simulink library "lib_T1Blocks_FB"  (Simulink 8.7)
settings: Solver=ode3  SolverMode=SingleTasking  StartTime=0.0  StopTime=1  FixedStep=0.02/16384  RelTol=1e-3
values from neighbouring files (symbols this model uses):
  Tstep = 0.0005    [TestOrthOscObjO_init.m]    (also in TestWaveMng_init.m = 5e-05)
undefined symbols (not defined in the file or in its folder): lim, max_error, min_decrease, min_reset, P_TA, T1, Td, y0
libraries: lib_T1Blocks_FB x7, simulink x2

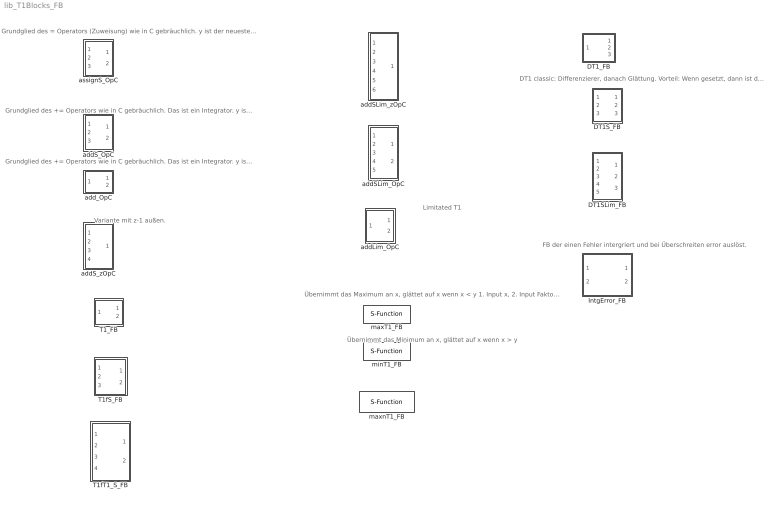
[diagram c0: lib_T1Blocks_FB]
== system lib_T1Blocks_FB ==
  note: Limitated T1
  note: Variante mit z-1 außen.
  note: Übernimmt das Maximum an x, glättet auf x wenn x < y 1. Input x, 2. Input Faktor zum Glätten
  note: DT1 classic: Differenzierer, danach Glättung. Vorteil: Wenn gesetzt, dann ist das Differnzial 0
  note: Grundglied des += Operators wie in C gebräuchlich. Das ist ein Integrator. y ist der neueste Wert. yz ist der gespeicherte Wert (Abarbeitung bevor +=). Setzen: Wird in C häufig an anderer Stelle ausgeführt.
  note: Grundglied des += Operators wie in C gebräuchlich. Das ist ein Integrator. y ist der neueste Wert. yz ist der gespeicherte Wert (Abarbeitung bevor +=). Ohne Setz-Möglichkeit. Initialwert als Parameter.
  note: FB der einen Fehler intergriert und bei Überschreiten error auslöst.
  note: Grundglied des = Operators (Zuweisung) wie in C gebräuchlich. y ist der neueste Wert, entweder =X oder =XS. yz ist der gespeicherte Wert. Setzen: Wird in C häufig an anderer Stelle ausgeführt.
  note: Übernimmt das Minimum an x, glättet auf x wenn x > y
  DT1SLim_FB : Subsystem
  DT1S_FB : Subsystem
  DT1_FB : Subsystem
  IntgError_FB : Subsystem
  T1_FB : Subsystem
  T1fS_FB : Subsystem
  T1fT1_S_FB : Subsystem
  addLim_OpC : Subsystem
  addSLim_OpC : Subsystem
  addSLim_zOpC : Subsystem
  addS_OpC : Subsystem
  addS_zOpC : Subsystem
  add_OpC : Subsystem
  assignS_OpC : Subsystem
  maxT1_FB : S-Function  FunctionName=maxT1_FB  Parameters=SampleTime  SFunctionDeploymentMode=off  EnableBusSupport=off
  maxnT1_FB : S-Function  FunctionName=maxnT1_FB  Parameters=SampleTime  SFunctionDeploymentMode=off  EnableBusSupport=off
  minT1_FB : S-Function  FunctionName=minT1_FB  Parameters=SampleTime  SFunctionDeploymentMode=off  EnableBusSupport=off

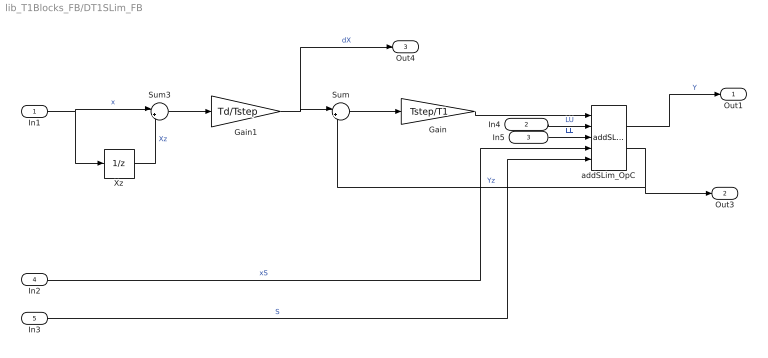
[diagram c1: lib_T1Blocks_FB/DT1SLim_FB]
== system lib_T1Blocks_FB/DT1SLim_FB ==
  In1 : Inport
  In4 : Inport  Port=2
  In5 : Inport  Port=3
  In2 : Inport  Port=4
  In3 : Inport  Port=5
  Gain : Gain  Gain=Tstep/T1
  Gain1 : Gain  Gain=Td/Tstep
  Sum : Sum  Inputs=|+-
  Sum3 : Sum  Inputs=|+-
  Xz : UnitDelay  SampleTime=-1
  addSLim_OpC : lib_T1Blocks_FB/addSLim_OpC
  Out1 : Outport
  Out3 : Outport  Port=2
  Out4 : Outport  Port=3
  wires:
  addSLim_OpC/2 -> Out3/1, Sum/2  "Yz"
  In3/1 -> addSLim_OpC/5  "S"
  In2/1 -> addSLim_OpC/4  "xS"
  Sum3/1 -> Gain1/1
  Xz/1 -> Sum3/2  "Xz"
  Gain1/1 -> Sum/1, Out4/1  "dX"
  addSLim_OpC/1 -> Out1/1  "Y"
  In1/1 -> Sum3/1, Xz/1  "x"
  Sum/1 -> Gain/1
  Gain/1 -> addSLim_OpC/1
  In4/1 -> addSLim_OpC/2  "LU"
  In5/1 -> addSLim_OpC/3  "LL"

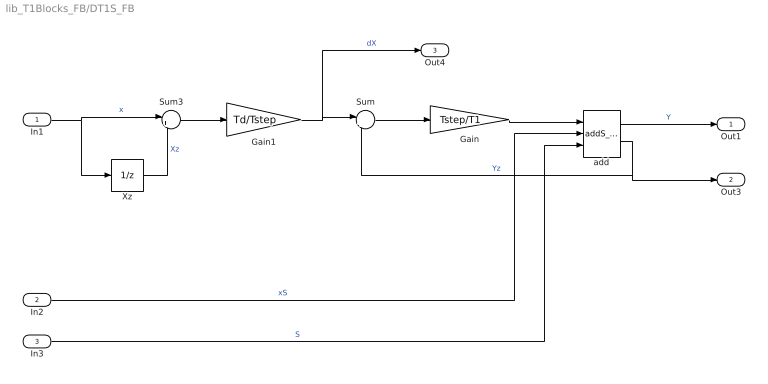
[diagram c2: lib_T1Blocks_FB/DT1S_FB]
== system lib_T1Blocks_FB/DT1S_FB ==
  In1 : Inport
  In2 : Inport  Port=2
  In3 : Inport  Port=3
  Gain : Gain  Gain=Tstep/T1
  Gain1 : Gain  Gain=Td/Tstep
  Sum : Sum  Inputs=|+-
  Sum3 : Sum  Inputs=|+-
  Xz : UnitDelay  SampleTime=-1
  add : lib_T1Blocks_FB/addS_OpC
  Out1 : Outport
  Out3 : Outport  Port=2
  Out4 : Outport  Port=3
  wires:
  Gain/1 -> add/1
  Sum/1 -> Gain/1
  In1/1 -> Xz/1, Sum3/1  "x"
  add/1 -> Out1/1  "Y"
  Gain1/1 -> Out4/1, Sum/1  "dX"
  Xz/1 -> Sum3/2  "Xz"
  Sum3/1 -> Gain1/1
  In2/1 -> add/2  "xS"
  In3/1 -> add/3  "S"
  add/2 -> Sum/2, Out3/1  "Yz"

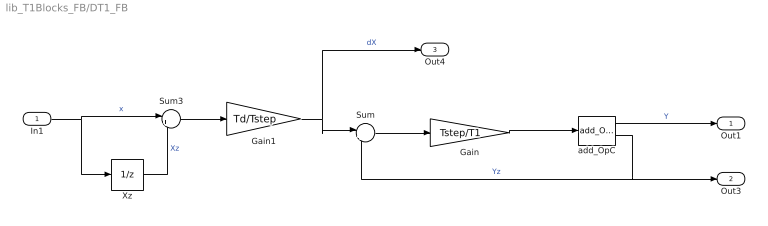
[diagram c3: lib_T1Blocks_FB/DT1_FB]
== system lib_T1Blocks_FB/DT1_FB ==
  In1 : Inport
  Gain : Gain  Gain=Tstep/T1
  Gain1 : Gain  Gain=Td/Tstep
  Sum : Sum  Inputs=|+-
  Sum3 : Sum  Inputs=|+-
  Xz : UnitDelay  SampleTime=-1
  add_OpC : lib_T1Blocks_FB/add_OpC  y0=0
  Out1 : Outport
  Out3 : Outport  Port=2
  Out4 : Outport  Port=3
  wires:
  add_OpC/2 -> Out3/1, Sum/2  "Yz"
  Sum3/1 -> Gain1/1
  Xz/1 -> Sum3/2  "Xz"
  Gain1/1 -> Sum/1, Out4/1  "dX"
  add_OpC/1 -> Out1/1  "Y"
  In1/1 -> Sum3/1, Xz/1  "x"
  Sum/1 -> Gain/1
  Gain/1 -> add_OpC/1

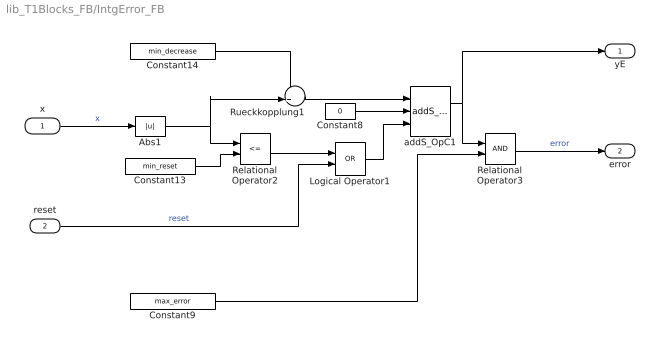
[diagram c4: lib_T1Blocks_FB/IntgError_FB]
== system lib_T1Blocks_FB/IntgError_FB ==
  x : Inport
  reset : Inport  Port=2
  Abs1 : Abs
  Constant13 : Constant  Value=min_reset  OutDataTypeStr=single
  Constant14 : Constant  Value=min_decrease  OutDataTypeStr=single
  Constant8 : Constant  Value=0  OutDataTypeStr=single
  Constant9 : Constant  Value=max_error  OutDataTypeStr=single
  Logical Operator1 : Logic  Operator=OR  AllPortsSameDT=off  OutDataTypeStr=boolean
  Relational Operator2 : RelationalOperator  Operator=<=  OutDataTypeStr=boolean
  Relational Operator3 : RelationalOperator  OutDataTypeStr=boolean
  Rueckkopplung1 : Sum  Inputs=++|
  addS_OpC1 : lib_T1Blocks_FB/addS_OpC
  yE : Outport
  error : Outport  Port=2
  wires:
  addS_OpC1/1 -> yE/1, Relational Operator3/1
  Constant9/1 -> Relational Operator3/2
  reset/1 -> Logical Operator1/2  "reset"
  x/1 -> Abs1/1  "x"
  Relational Operator3/1 -> error/1  "error"
  Relational Operator2/1 -> Logical Operator1/1
  Constant13/1 -> Relational Operator2/2
  Rueckkopplung1/1 -> addS_OpC1/1
  Constant14/1 -> Rueckkopplung1/1
  Logical Operator1/1 -> addS_OpC1/3
  Constant8/1 -> addS_OpC1/2
  Abs1/1 -> Rueckkopplung1/2, Relational Operator2/1

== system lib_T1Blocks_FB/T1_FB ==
  In1 : Inport
  Gain : Gain  Gain=P_TA/T1
  Sum : Sum  Inputs=|+-
  add_OpC : lib_T1Blocks_FB/add_OpC  y0=y0
  Out1 : Outport
  Out2 : Outport  Port=2
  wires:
  Gain/1 -> add_OpC/1
  Sum/1 -> Gain/1
  In1/1 -> Sum/1  "X"
  add_OpC/1 -> Out1/1  "Y"
  add_OpC/2 -> Out2/1, Sum/2  "Yz"

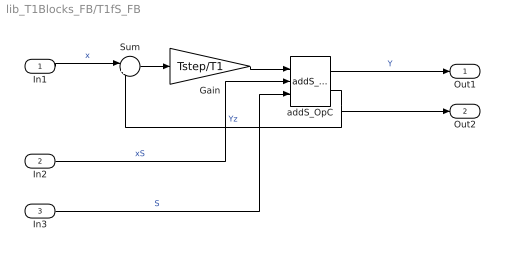
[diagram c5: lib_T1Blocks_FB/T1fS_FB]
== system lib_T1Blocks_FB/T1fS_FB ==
  In1 : Inport
  In2 : Inport  Port=2
  In3 : Inport  Port=3  OutDataTypeStr=boolean
  Gain : Gain  Gain=Tstep/T1
  Sum : Sum  Inputs=|+-
  addS_OpC : lib_T1Blocks_FB/addS_OpC
  Out1 : Outport
  Out2 : Outport  Port=2
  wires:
  Gain/1 -> addS_OpC/1
  Sum/1 -> Gain/1
  In1/1 -> Sum/1  "x"
  addS_OpC/1 -> Out1/1  "Y"
  addS_OpC/2 -> Out2/1, Sum/2  "Yz"
  In2/1 -> addS_OpC/2  "xS"
  In3/1 -> addS_OpC/3  "S"

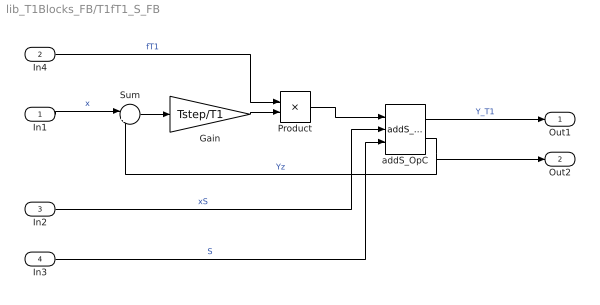
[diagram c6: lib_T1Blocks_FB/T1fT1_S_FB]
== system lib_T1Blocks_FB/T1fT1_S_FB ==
  In1 : Inport
  In4 : Inport  Port=2
  In2 : Inport  Port=3
  In3 : Inport  Port=4  OutDataTypeStr=boolean
  Gain : Gain  Gain=Tstep/T1
  Product : Product
  Sum : Sum  Inputs=|+-
  addS_OpC : lib_T1Blocks_FB/addS_OpC
  Out1 : Outport
  Out2 : Outport  Port=2
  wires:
  In3/1 -> addS_OpC/3  "S"
  In2/1 -> addS_OpC/2  "xS"
  addS_OpC/2 -> Sum/2, Out2/1  "Yz"
  addS_OpC/1 -> Out1/1  "Y_T1"
  In1/1 -> Sum/1  "x"
  Sum/1 -> Gain/1
  Product/1 -> addS_OpC/1
  In4/1 -> Product/1  "fT1"
  Gain/1 -> Product/2

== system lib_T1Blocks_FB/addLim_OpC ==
  x : Inport
  Delay : Delay  DelayLength=1
  Saturation : Saturate  UpperLimit=lim  LowerLimit=-lim
  Sum6 : Sum  Inputs=|++
  y : Outport
  yz : Outport  Port=2
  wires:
  Saturation/1 -> Sum6/2
  Delay/1 -> yz/1, Saturation/1
  x/1 -> Sum6/1
  Sum6/1 -> y/1, Delay/1

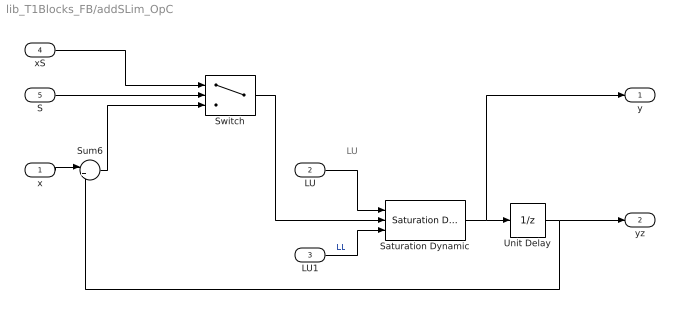
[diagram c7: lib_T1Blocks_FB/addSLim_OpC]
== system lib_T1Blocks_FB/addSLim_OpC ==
  note: LU
  x : Inport
  LU : Inport  Port=2
  LU1 : Inport  Port=3
  xS : Inport  Port=4
  S : Inport  Port=5  OutDataTypeStr=boolean
  Saturation Dynamic : simulink/Discontinuities/Saturation Dynamic  OutMin=[]  OutMax=[]  OutDataTypeStr=Inherit: Same as second input  OutDataType=fixdt(1, 16)  OutScaling=2^-10  DoSatur=off
  Sum6 : Sum  Inputs=|++
  Switch : Switch  Criteria=u2 ~= 0
  Unit Delay : UnitDelay  SampleTime=-1
  y : Outport
  yz : Outport  Port=2
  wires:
  Switch/1 -> Saturation Dynamic/2
  S/1 -> Switch/2
  Unit Delay/1 -> yz/1, Sum6/2
  xS/1 -> Switch/1
  x/1 -> Sum6/1
  Sum6/1 -> Switch/3
  Saturation Dynamic/1 -> y/1, Unit Delay/1
  LU/1 -> Saturation Dynamic/1
  LU1/1 -> Saturation Dynamic/3  "LL"

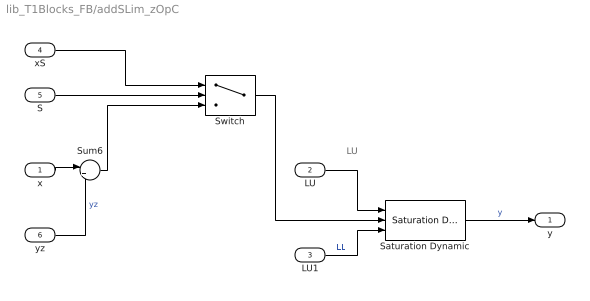
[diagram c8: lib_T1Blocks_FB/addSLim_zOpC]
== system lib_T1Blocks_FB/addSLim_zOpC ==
  note: LU
  x : Inport
  LU : Inport  Port=2
  LU1 : Inport  Port=3
  xS : Inport  Port=4
  S : Inport  Port=5  OutDataTypeStr=boolean
  yz : Inport  Port=6
  Saturation Dynamic : simulink/Discontinuities/Saturation Dynamic  OutMin=[]  OutMax=[]  OutDataTypeStr=Inherit: Same as second input  OutDataType=fixdt(1, 16)  OutScaling=2^-10  DoSatur=off
  Sum6 : Sum  Inputs=|++
  Switch : Switch  Criteria=u2 ~= 0
  y : Outport
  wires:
  LU1/1 -> Saturation Dynamic/3  "LL"
  LU/1 -> Saturation Dynamic/1
  Saturation Dynamic/1 -> y/1  "y"
  Sum6/1 -> Switch/3
  x/1 -> Sum6/1
  xS/1 -> Switch/1
  S/1 -> Switch/2
  Switch/1 -> Saturation Dynamic/2
  yz/1 -> Sum6/2  "yz"

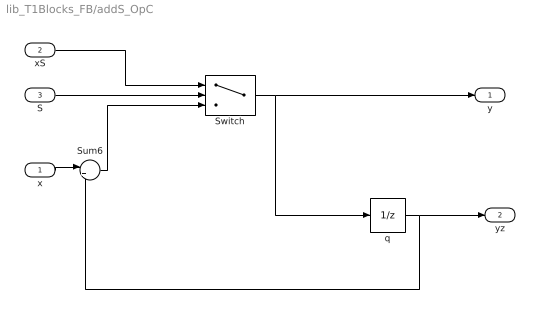
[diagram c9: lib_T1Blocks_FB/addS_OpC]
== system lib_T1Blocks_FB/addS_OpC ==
  x : Inport
  xS : Inport  Port=2
  S : Inport  Port=3  OutDataTypeStr=boolean
  Sum6 : Sum  Inputs=|++
  Switch : Switch  Criteria=u2 ~= 0
  q : UnitDelay  SampleTime=-1
  y : Outport
  yz : Outport  Port=2
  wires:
  Sum6/1 -> Switch/3
  x/1 -> Sum6/1
  xS/1 -> Switch/1
  q/1 -> Sum6/2, yz/1
  S/1 -> Switch/2
  Switch/1 -> q/1, y/1

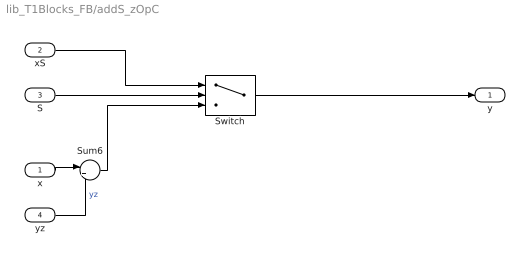
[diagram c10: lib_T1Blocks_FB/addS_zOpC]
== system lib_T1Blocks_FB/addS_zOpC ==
  x : Inport
  xS : Inport  Port=2
  S : Inport  Port=3  OutDataTypeStr=boolean
  yz : Inport  Port=4
  Sum6 : Sum  Inputs=|++
  Switch : Switch  Criteria=u2 ~= 0
  y : Outport
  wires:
  Switch/1 -> y/1
  S/1 -> Switch/2
  xS/1 -> Switch/1
  x/1 -> Sum6/1
  Sum6/1 -> Switch/3
  yz/1 -> Sum6/2  "yz"

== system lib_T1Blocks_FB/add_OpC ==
  x : Inport
  Delay : Delay  DelayLength=1  InitialCondition=y0
  Sum6 : Sum  Inputs=|++
  y : Outport
  yz : Outport  Port=2
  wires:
  Sum6/1 -> Delay/1, y/1
  x/1 -> Sum6/1
  Delay/1 -> Sum6/2, yz/1

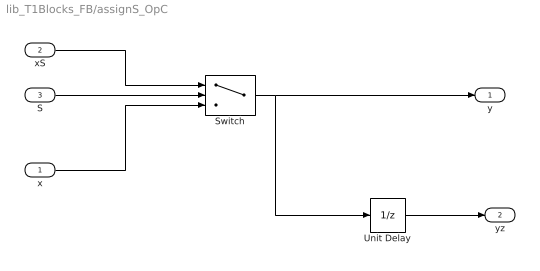
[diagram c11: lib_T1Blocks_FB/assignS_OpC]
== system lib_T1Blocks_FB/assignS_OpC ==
  x : Inport
  xS : Inport  Port=2
  S : Inport  Port=3  OutDataTypeStr=boolean
  Switch : Switch  Criteria=u2 ~= 0
  Unit Delay : UnitDelay  SampleTime=-1
  y : Outport
  yz : Outport  Port=2
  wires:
  Switch/1 -> y/1, Unit Delay/1
  S/1 -> Switch/2
  Unit Delay/1 -> yz/1
  xS/1 -> Switch/1
  x/1 -> Switch/3
